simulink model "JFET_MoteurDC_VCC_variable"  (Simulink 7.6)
settings: Solver=ode15s  StartTime=0.0  StopTime=30  RelTol=1e-3
StopFcn:
  | clc, close all
  | load signaux_VI.mat
  | plotyy(x(1,:),x(2,:), x(1,:),x(3,:))
  | grid
  | title('Tension d''alimentation Vcc et courant de drain Id')
  | xlabel('temps')
  | 
  | load signaux_VitPos.mat
  | figure
  | plotyy(y(1,:),y(2,:), y(1,:),y(3,:))
  | grid
  | title('Vitesse (rad/s) et Position (rad) de l''arbre moteur')
  | xlabel('temps')
libraries: fl_lib x15, nesl_utility x6, elec_lib x4

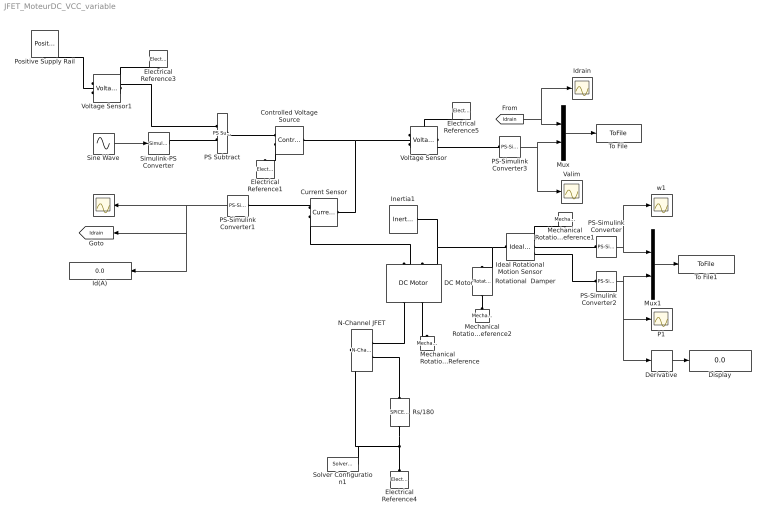
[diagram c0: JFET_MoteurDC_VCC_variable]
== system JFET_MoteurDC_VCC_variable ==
  Controlled Voltage Source : fl_lib/Electrical/Electrical Sources/Controlled Voltage Source  DialogController=NetworkEngine.DynNeDlgSource  SystemSampleTime=-1  i_Log=off  v_Log=off  LocalVarNames=|i|v  LocalVarDescs=|i|v  LocalVarLogging=[0 0]
  Current Sensor : fl_lib/Electrical/Electrical Sensors/Current Sensor  DialogController=NetworkEngine.DynNeDlgSource  SystemSampleTime=-1  i1_Log=off  v1_Log=off  LocalVarNames=|i1|v1  LocalVarDescs=|i1|v1  LocalVarLogging=[0 0]
  DC Motor : elec_lib/Actuators & Drivers/Rotational Actuators/DC Motor  DialogController=NetworkEngine.DynNeDlgSource  SystemSampleTime=-1  parameterization=1  Ra=3.9 Ohm  La=1.2e-05 H  emf_or_torque=1  Kv=7.2e-05 V/rpm  Ki=6.876e-04 N*m/A  T_stall=2.4e-04 N*m  w_max=1.91e+04 rpm  w_rated=1.5e+04 rpm  P_rated=0.08 W  V_rated=1.5 V  J=0.01 g*cm^2  lam=1e-08 N*m/(rad/s)  speed0=0 rpm  current_Log=off  voltage_Log=off  power_Log=off  i2r_Log=off  torque_Log=off  speed_Log=off  LocalVarNames=|current|voltage|power|i2r|torque|speed  LocalVarDescs=|Current (A)|Voltage (V)|Power (W)|Electrical losses (W)|Torque (Nm)|Angular speed (rad/s)  LocalVarLogging=[0 0 0 0 0 0]
  Derivative : Derivative
  Display : Display
  Electrical Reference{1,3..5} (4 alike) : fl_lib/Electrical/Electrical Elements/Electrical Reference  DialogController=NetworkEngine.DynNeDlgSource  SystemSampleTime=-1  i_Log=off  LocalVarNames=|i  LocalVarDescs=|i  LocalVarLogging=[]
  I : Scope
  Id(A) : Display
  Ideal Rotational Motion Sensor : fl_lib/Mechanical/Mechanical Sensors/Ideal Rotational Motion Sensor  DialogController=NetworkEngine.DynNeDlgSource  SystemSampleTime=-1  offset=0 rad  w_Log=off  t_Log=off  phi_Log=off  LocalVarNames=|w|t|phi  LocalVarDescs=|w|t|phi  LocalVarLogging=[0 0 0]
  Idrain : Scope
  Inertia1 : fl_lib/Mechanical/Rotational Elements/Inertia  DialogController=NetworkEngine.DynNeDlgSource  SystemSampleTime=-1  inertia=1e-7 kg*m^2  initial_velocity=0 rad/s  t_Log=off  LocalVarNames=|t  LocalVarDescs=|t  LocalVarLogging=0
  Mechanical Rotational Reference : fl_lib/Mechanical/Rotational Elements/Mechanical Rotational Reference  DialogController=NetworkEngine.DynNeDlgSource  SystemSampleTime=-1  t_Log=off  LocalVarNames=|t  LocalVarDescs=|t  LocalVarLogging=0
  Mechanical Rotational Reference1 : fl_lib/Mechanical/Rotational Elements/Mechanical Rotational Reference  DialogController=NetworkEngine.DynNeDlgSource  SystemSampleTime=-1  t_Log=off  LocalVarNames=|t  LocalVarDescs=|t  LocalVarLogging=0
  Mechanical Rotational Reference2 : fl_lib/Mechanical/Rotational Elements/Mechanical Rotational Reference  DialogController=NetworkEngine.DynNeDlgSource  SystemSampleTime=-1  t_Log=off  LocalVarNames=|t  LocalVarDescs=|t  LocalVarLogging=0
  Mux : Mux  Inputs=2
  Mux1 : Mux  Inputs=2
  N-Channel JFET : elec_lib/Semiconductor Devices/N-Channel JFET  DialogController=NetworkEngine.DynNeDlgSource  SystemSampleTime=-1  parameterization=1  Igss=-1 nA  Idss=17 mA  Idss_v="[  0 15 ] V"  ssig="[  3e+03 10 ] uS"  ssig_v="[  0 15 ] V"  Beta=1e-04 A/V^2  IS=1e-14 A  Tmeas=25 C  Vt0=-2 V  Lchannel=0 1/V  RS=0.1 Ohm  RD=0.1 Ohm  C_param=1  C_GS=3 pF  C_GD=1.5 pF  C_iss=4.5 pF  C_rss=1.5 pF  LocalVarLogging=[]
  P1 : Scope
  PS Subtract : fl_lib/Physical Signals/Functions/PS Subtract  DialogController=NetworkEngine.DynNeDlgSource  SystemSampleTime=-1  LocalVarLogging=[]
  PS-Simulink Converter{,1..3} (4 alike) : nesl_utility/PS-Simulink Converter  DialogController=NetworkEngine.DynNeUtilDlgSource  SystemSampleTime=-1  PhysicalDomain=network_engine_domain  LeftPortType=input  RightPortType=output  SubClassName=ps_output  Unit=1  AffineConversion=off
  Positive Supply Rail : elec_lib/Sources/Positive Supply Rail  DialogController=NetworkEngine.DynNeDlgSource  SystemSampleTime=-1  v0=15 V  current_Log=off  voltage_Log=off  power_Log=off  LocalVarNames=|current|voltage|power  LocalVarDescs=|Current (A)|Voltage (V)|Power (W)  LocalVarLogging=[0 0 0]
  Rotational  Damper : fl_lib/Mechanical/Rotational Elements/Rotational Damper  DialogController=NetworkEngine.DynNeDlgSource  SystemSampleTime=-1  D=1e-8 N*m/(rad/s)  t_Log=off  w_Log=off  LocalVarNames=|t|w  LocalVarDescs=|t|w  LocalVarLogging=[0 0]
  Rs/180 : elec_lib/Additional Components/SPICE-Compatible Components/Passive Devices/SPICE Resistor  DialogController=NetworkEngine.DynNeDlgSource  SystemSampleTime=-1  SCALE=1  R_param=1  R=180 Ohm  RSH=0 Ohm  LENGTH=1e-06 m  WIDTH=1e-06 m  NARROW=0 m  T_param=1  TC1=0 1/K  TC2=0 1/K^2  TOFFSET=0 K  TFIXED=300.15 K  TMEAS=300.15 K  LocalVarLogging=[]
  Simulink-PS Converter : nesl_utility/Simulink-PS Converter  DialogController=NetworkEngine.DynNeUtilDlgSource  SystemSampleTime=-1  PhysicalDomain=network_engine_domain  LeftPortType=input  RightPortType=output  SubClassName=ps_input  Unit=1  AffineConversion=off  InputFilterTimeConstant=.001  UdotUserProvided=0
  Sine Wave : Sin  Amplitude=5  Frequency=0.5  SampleTime=0
  Solver Configuration1 : nesl_utility/Solver Configuration  DialogController=NetworkEngine.DynNeUtilDlgSource  SystemSampleTime=-1  PhysicalDomain=network_engine_domain  LeftPortType=input  RightPortType=generic  SubClassName=solver  Accelerate=off  Profile=off  ResidualTolerance=1e-9  MaxNonlinIter=12  MaxModeIter=2  DoFixedCost=off  UseLocalSampling=off  DoDC=off  LinearAlgebra=Sparse  LocalSolverSampleTime=.001  LocalSolverChoice=NE_BACKWARD_EULER_ADVANCER  UseLocalSolver=off
  To File : ToFile  Filename=signaux_VI  MatrixName=x
  To File1 : ToFile  Filename=signaux_VitPos  MatrixName=y
  Valim : Scope
  Voltage Sensor : fl_lib/Electrical/Electrical Sensors/Voltage Sensor  DialogController=NetworkEngine.DynNeDlgSource  SystemSampleTime=-1  i1_Log=off  v1_Log=off  LocalVarNames=|i1|v1  LocalVarDescs=|i1|v1  LocalVarLogging=[0 0]
  Voltage Sensor1 : fl_lib/Electrical/Electrical Sensors/Voltage Sensor  DialogController=NetworkEngine.DynNeDlgSource  SystemSampleTime=-1  i1_Log=off  v1_Log=off  LocalVarNames=|i1|v1  LocalVarDescs=|i1|v1  LocalVarLogging=[0 0]
  w1 : Scope
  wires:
  PS-Simulink Converter/1 -> Mux1/1, w1/1
  Sine Wave/1 -> Simulink-PS Converter/1
  PS-Simulink Converter1/1 -> I/1, [Idrain], Id(A)/1
  PS-Simulink Converter2/1 -> Mux1/2, P1/1, Derivative/1
  PS-Simulink Converter3/1 -> Mux/2, Valim/1
  Mux/1 -> To File/1
  [Idrain] -> Mux/1, Idrain/1
  Mux1/1 -> To File1/1
  Derivative/1 -> Display/1
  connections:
  Rs/180/LConn1 -- N-Channel JFET/RConn2
  DC Motor/RConn1 -- N-Channel JFET/RConn1
  Rs/180/RConn1 -- N-Channel JFET/LConn1 -- Solver Configuration1/RConn1 -- Electrical Reference4/LConn1
  Voltage Sensor/RConn1 -- PS-Simulink Converter3/LConn1
  Voltage Sensor/RConn2 -- Electrical Reference5/LConn1
  DC Motor/RConn2 -- Mechanical Rotational Reference/LConn1
  Ideal Rotational Motion Sensor/RConn2 -- PS-Simulink Converter/LConn1
  Ideal Rotational Motion Sensor/RConn1 -- Mechanical Rotational Reference1/LConn1
  Ideal Rotational Motion Sensor/LConn1 -- DC Motor/LConn2 -- Inertia1/LConn1 -- Rotational  Damper/LConn1
  Voltage Sensor1/LConn1 -- Positive Supply Rail/RConn1
  Voltage Sensor1/RConn1 -- PS Subtract/LConn1
  Controlled Voltage Source/RConn2 -- Electrical Reference1/LConn1
  Voltage Sensor1/RConn2 -- Electrical Reference3/LConn1
  Simulink-PS Converter/RConn1 -- PS Subtract/LConn2
  PS Subtract/RConn1 -- Controlled Voltage Source/RConn1
  Current Sensor/RConn1 -- PS-Simulink Converter1/LConn1
  Current Sensor/RConn2 -- DC Motor/LConn1
  Controlled Voltage Source/LConn1 -- Voltage Sensor/LConn1 -- Current Sensor/LConn1
  Ideal Rotational Motion Sensor/RConn3 -- PS-Simulink Converter2/LConn1
  Rotational  Damper/RConn1 -- Mechanical Rotational Reference2/LConn1
